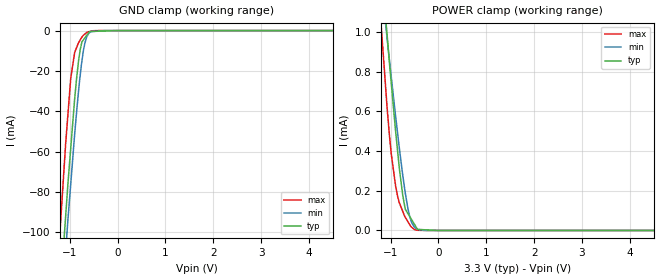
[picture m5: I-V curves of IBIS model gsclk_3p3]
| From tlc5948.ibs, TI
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|   gsclk_3p3 Model
[Model]   gsclk_3p3
Model_type   Input
Vinl = 0.99
Vinh = 2.31
|   typ   min   max
|   (nom PVT)   (fast PVT)   (slow PVT)
|C_comp from frequency sweep method (F=33MHz)
|Average
|C_comp   8.184e-13   7.974e-13   8.823e-13
|C_comp from LC tank measurement(L=1nH)
|Average
|Resonant Frequency(Hz)   6.720e+09   6.850e+09   6.560e+09
C_comp   5.615e-13   5.404e-13   5.892e-13
| Where nom  PVT is Nominal Process, 3.3V, 90C
|   Fast PVT is Strong Process,  3.6V, -40C
|   Slow PVT is Weak Process,   3V, 150C
[Model Spec]
|Subparameter   typ   min   max
Vinl   0.99   0.9   1.08
Vinh   2.31   2.1   2.52
[Voltage Range]   3.3   3   3.6
|Ambient Temperature   25   85   -40
|Junction Temperature
[Temperature Range]   90   150   -40
[Power Clamp Reference]   3.3   3   3.6
[GND Clamp Reference]   0   0   0
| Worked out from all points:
|   GND clamp passes 1 mA (typ) near -0.60 V on its own axis
|   POWER clamp passes 1 mA (typ) near -1.08 V on its own axis
[GND Clamp]
|   Voltage   I(typ)   I(min)   I(max)
-3.3V     -951.6mA   -928.2mA   -1.005A
-1.215V   -136mA     -152.1mA   -103.9mA
-1.084V   -91.56mA   -109mA     -55.62mA
-1.038V   -76.14mA   -94mA      -41.71mA
-979.2mV  -58.48mA   -76.26mA   -23.78mA
-896.4mV  -33.78mA   -51.31mA   -10.8mA
-815.1mV  -15mA      -30.02mA   -6.071mA
-745.8mV  -5.612mA   -15.23mA   -3.285mA
-720mV    -4.789mA   -10.81mA   -2.463mA
-637.2mV  -2.146mA   -2.795mA   -782.3uA
-285mV    -221.9uA   -4.709uA   -7.129uA
6.6V      0A         0A         0A
[POWER Clamp]
|   Voltage   I(typ)   I(min)   I(max)
-3.3V     7.852mA    6.423mA    9.069mA
-1.213V   1.39mA     1.29mA     1.087mA
-1.171V   1.267mA    1.194mA    947.7uA
-1.076V   995.2uA    976.9uA    630.4uA
-986.4mV  743.2uA    775.1uA    386.6uA
-896.4mV  502.3uA    578.5uA    226uA
-745.8mV  176.7uA    278.4uA    96.06uA
-693mV    106.9uA    188.3uA    66.25uA
-636mV    84.37uA    108.4uA    43.52uA
-504mV    32.11uA    17.53uA    5.325uA
-3.3mV    0A         18.73nA    0A
6.6V      0A         0A         0A
